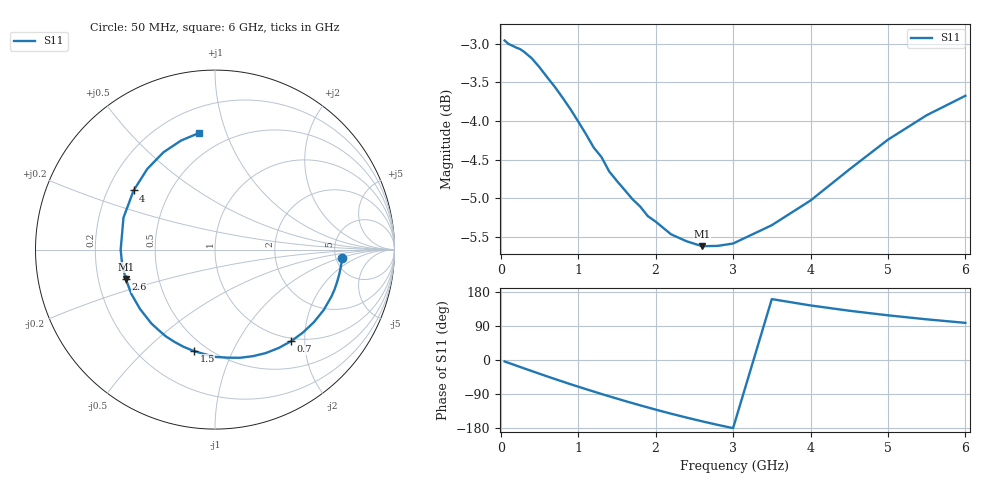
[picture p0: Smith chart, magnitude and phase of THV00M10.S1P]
! SIEMENS Discrete & RF Semiconductors
! BAS70
! Si Schottky Diode in SOT23
! IF = 0.1 mA
! S-Parameters:  February  1997
# GHz  S  MA  R  50
!  f  S11
! GHz  MAG  ANG
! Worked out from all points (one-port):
!   34 points, 50 MHz to 6 GHz, reference 50 ohm
!   lowest |S11| = -5.6 dB at 2.6 GHz (marker M1), VSWR 3.20, Z = 16 - j7.21 ohm
!   |S11| at or under -10 dB: nowhere
!   S11 on the Smith chart (normalised r, x): 50 MHz: 5.71, -1.09; 700 MHz: 0.95, -1.73; 1.5 GHz: 0.43, -0.72; 2.6 GHz: 0.32, -0.14; 4 GHz: 0.31, +0.30; 6 GHz: 0.35, +0.81
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0.05  0.7114 -3.8
0.15  0.7059 -11.1
0.25  0.7023 -18.3
0.3  0.6995 -22.0
0.4  0.6927 -29.1
0.5  0.6836 -36.2
0.6  0.6734 -43.3
0.7  0.6637 -50.2
0.8  0.6531 -57.0
0.9  0.6422 -63.8
1  0.6305 -70.3
1.1  0.6188 -76.9
1.3  0.598 -89.6
1.5  0.577 -101.8
1.6  0.5693 -107.9
1.8  0.5555 -119.6
2  0.5431 -130.9
2.2  0.5329 -141.7
2.4  0.5274 -152.0
2.6  0.5236 -161.8
2.8  0.5238 -171.1
3  0.5256 -179.9
3.5  0.5402 160.7
4  0.5604 144.0
4.5  0.5869 130.0
5  0.6136 117.9
5.5  0.6364 107.3
6  0.6551 98.0
